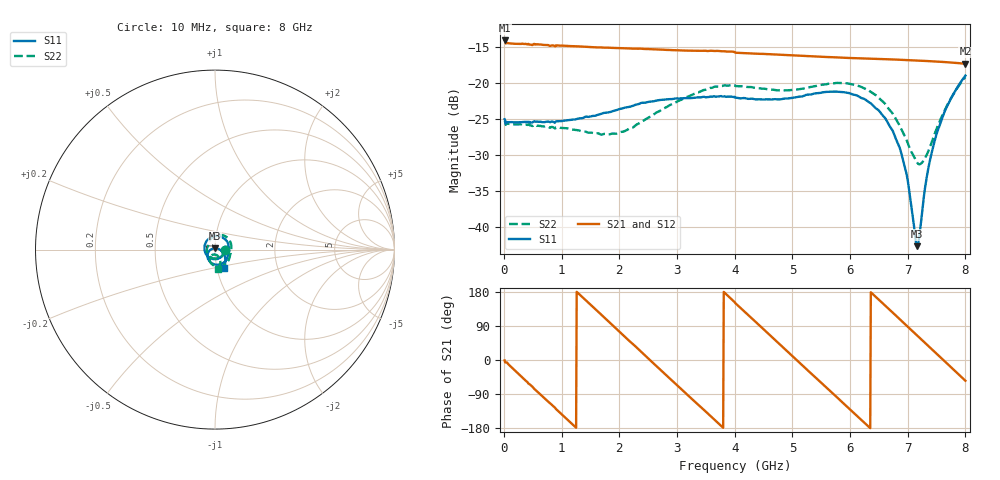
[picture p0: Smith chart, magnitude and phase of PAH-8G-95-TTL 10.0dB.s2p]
! MTS Systemtechnik GmbH
! S-Parameters
! Model: PAH-8G/95-TTL
! Attenuation Step: 10.0dB
! Rohde & Schwarz ZVB8 2Ports - Version 4.11 - 1145.1010k08 SN: 100119
! S2P File Measurements:
! S11 S21 S12 S22
# HZ  S  DB  R  50.00
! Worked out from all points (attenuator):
!   800 points, 10 MHz to 8 GHz, reference 50 ohm
!   highest |S21| = -14.05 dB at 10 MHz (marker M1); lowest = -17.3 dB at 8 GHz (marker M2)
!   lowest |S11| = -42.7 dB at 7.16 GHz (marker M3), VSWR 1.01, Z = 49.9 + j0.724 ohm
!   |S11| at or under -10 dB: start of sweep to end of sweep
!   |S22| runs from -31.3 to -19.2 dB; largest |S21 - S12| = 0.0027
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1e7  -25.04 -3.3  -14.05 -1.2  -13.96 -1.1  -25.25 -3.5
6.4e8  -25.40 -81.4  -14.62 -92.2  -14.61 -92.2  -25.99 -88.2
1.03e9  -25.24 -128.9  -14.78 -147.5  -14.78 -147.5  -26.29 -136.9
1.35e9  -24.91 -163.9  -14.91 167.1  -14.91 167.2  -26.73 -170.1
1.96e9  -23.74 141.8  -15.11 80.2  -15.13 80.3  -27.02 147.4
2.36e9  -22.82 112.8  -15.19 24.4  -15.19 24.4  -25.52 129.9
2.68e9  -22.38 91.6  -15.32 -21.4  -15.31 -21.2  -23.97 113.3
3.28e9  -22.07 56.5  -15.48 -106.0  -15.50 -106.4  -21.56 76.4
3.68e9  -21.91 37.3  -15.51 -161.7  -15.48 -161.3  -20.47 51.2
4.01e9  -22.03 20.9  -15.76 150.2  -15.76 150.0  -20.41 29.7
4.57e9  -22.26 -3.3  -15.96 71.0  -15.98 71.0  -20.88 0.1
4.97e9  -22.09 -20.1  -16.11 14.4  -16.12 14.3  -20.97 -17.1
5.34e9  -21.55 -38.3  -16.26 -37.5  -16.27 -37.6  -20.52 -33.1
5.87e9  -21.24 -73.7  -16.45 -112.2  -16.47 -112.2  -20.01 -63.8
6.28e9  -22.39 -107.6  -16.58 -170.0  -16.60 -170.1  -20.85 -91.7
6.67e9  -25.76 -144.4  -16.68 134.9  -16.69 134.9  -23.60 -116.0
6.95e9  -31.69 -177.3  -16.78 95.0  -16.79 95.0  -27.40 -123.2
7.16e9  -42.74 96.4  -16.86 65.1  -16.86 65.1  -31.03 -103.8
7.2e9  -41.41 58.7  -16.87 59.4  -16.88 59.4  -31.32 -97.3
7.35e9  -32.20 3.1  -16.93 38.1  -16.94 38.0  -29.63 -71.5
7.49e9  -27.37 -16.4  -16.99 18.1  -17.00 18.1  -26.58 -62.7
8e9  -18.96 -64.1  -17.30 -54.7  -17.31 -54.7  -19.17 -80.4
